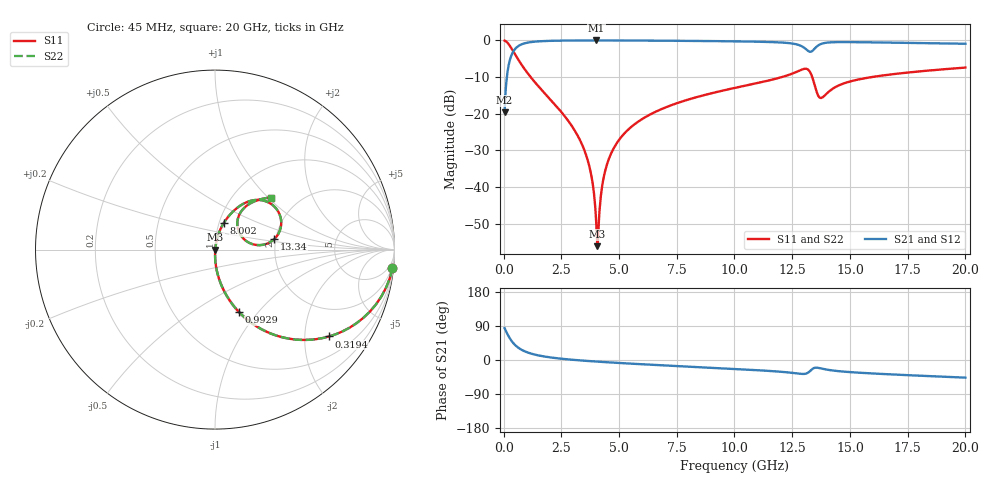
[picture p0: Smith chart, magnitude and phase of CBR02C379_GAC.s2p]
! S-parameter model data by Modelithics Inc.  support@modelithics.com 813-866-6335  Tampa FL USA
! S-Parameter data specifications:
! Substrate: 20-mil Rogers 4350B, substrate thickness, H=0.508mm, Dielectric constant, Er=3.75
! PCB Mounting Pad Footprint: Pad width, PadW=0.32mm , Pad length, PadL=0.37mm , Pad gap, PadG (edge-to-edge)=0.19mm , Reference planes=0.93mm apart
#  GHz  S  MA  R 50
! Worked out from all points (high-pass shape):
!   801 points, 45 MHz to 20 GHz, reference 50 ohm
!   highest |S21| = -0.01 dB at 4.011 GHz (marker M1); lowest = -19.6 dB at 45 MHz (marker M2)
!   |S21| within 3 dB of the highest: 422.7 MHz to 13.23 GHz (12.81 GHz wide, 188 % of centre); 13.33 GHz to end of sweep
!   lowest |S11| = -56.1 dB at 4.061 GHz (marker M3), VSWR 1.00, Z = 50.2 - j0.0469 ohm
!   |S11| at or under -10 dB: 1.174 GHz to 12.05 GHz (10.88 GHz wide, 164 % of centre); 13.37 GHz to 15.94 GHz (2.568 GHz wide, 17.5 % of centre)
!   |S22| runs from -56.1 to 0.0 dB; largest |S21 - S12| = 0
!   S11 on the Smith chart (normalised r, x): 45 MHz: 1, -19; 319.4 MHz: 0.99, -2.64; 992.9 MHz: 0.99, -0.80; 8.002 GHz: 1.05, +0.32; 13.34 GHz: 1.96, +0.25; 20 GHz: 1.47, +1.04
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0.045  0.9945 -6.1  0.1048 83.9  0.1048 83.9  0.9945 -6.1
0.194662  0.9094 -24.8  0.4155 65.2  0.4155 65.2  0.9094 -24.8
0.319381  0.7988 -37.3  0.6011 52.7  0.6011 52.7  0.7988 -37.3
0.618706  0.5587 -56.6  0.8285 33.3  0.8285 33.3  0.5587 -56.6
0.992862  0.3748 -68.9  0.9261 21.0  0.9261 21.0  0.3748 -68.9
3.387462  0.03879 -89.3  0.9977 -1.4  0.9977 -1.4  0.03879 -89.3
3.786563  0.0152 -87.5  0.9983 -3.2  0.9983 -3.2  0.0152 -87.5
4.011056  0.003333 -66.9  0.9984 -4.1  0.9984 -4.1  0.003333 -66.9
4.060944  0.00157 -17.3  0.9984 -4.3  0.9984 -4.3  0.00157 -17.3
4.135775  0.003828 61.7  0.9984 -4.6  0.9984 -4.6  0.003828 61.7
4.360269  0.01478 78.4  0.9982 -5.5  0.9982 -5.5  0.01478 78.4
4.759369  0.03343 80.3  0.9977 -7.0  0.9977 -7.0  0.03343 80.3
5.507681  0.06533 78.9  0.9961 -9.6  0.9961 -9.6  0.06533 78.9
6.704981  0.111 75.5  0.9918 -13.5  0.9918 -13.5  0.111 75.5
8.002056  0.1564 71.7  0.9855 -17.5  0.9855 -17.5  0.1564 71.7
10.0225  0.2256 65.5  0.971 -23.7  0.971 -23.7  0.2256 65.5
12.74137  0.379 46.5  0.8746 -35.6  0.8746 -35.6  0.379 46.5
13.34002  0.334 9.9  0.7081 -25.3  0.7081 -25.3  0.334 9.9
13.36496  0.3179 8.3  0.7166 -24.0  0.7166 -24.0  0.3179 8.3
13.76406  0.1646 33.5  0.8982 -22.5  0.8982 -22.5  0.1646 33.5
16.68248  0.341 51.3  0.9336 -37.7  0.9336 -37.7  0.341 51.3
20  0.4262 42.9  0.9002 -46.6  0.9002 -46.6  0.4262 42.9
